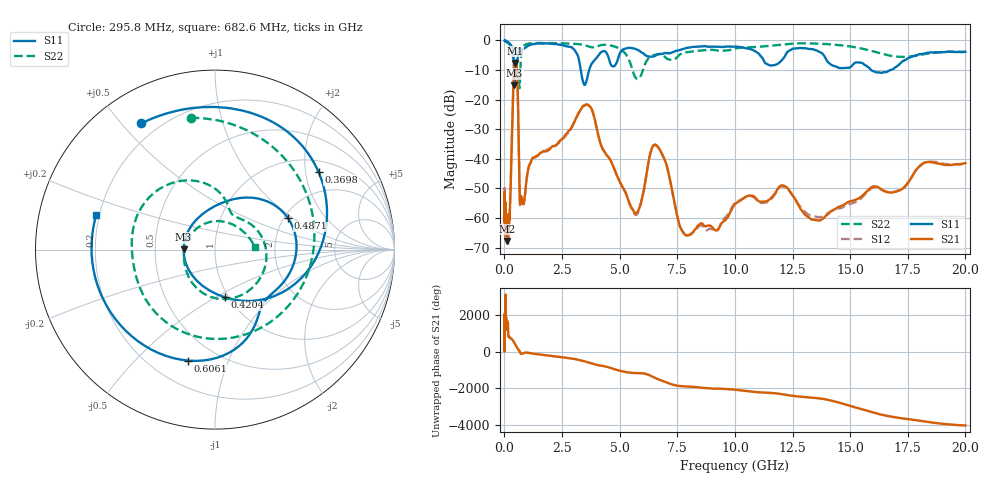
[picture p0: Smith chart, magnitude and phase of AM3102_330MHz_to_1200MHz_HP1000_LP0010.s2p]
! Date/Time: Tue, Sep 11, 2018 5:16 PM
! Network Analyzer: Agilent Technologies E8362B Rev: A.07.50.63
! Sweep from 0.010 to 20.000 GHz, 1601 Points, Sweep Type: LOG
! Power Supply: 4.949 V, 0.001 A
# Hz S DB R 50
!freq MagS11 AngS11 MagS21 AngS21 MagS12 AngS12 MagS22 AngS22
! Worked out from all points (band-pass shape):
!   1601 points, 10 MHz to 20 GHz, reference 50 ohm
!   highest |S21| = -7.59 dB at 455.8 MHz (marker M1); lowest = -67.8 dB at 118.3 MHz (marker M2)
!   |S21| within 3 dB of the highest: 411.3 MHz to 552.9 MHz (141.6 MHz wide, 29.4 % of centre)
!   lowest |S11| = -15.1 dB at 438.8 MHz (marker M3), VSWR 1.42, Z = 35.1 + j0.0801 ohm
!   |S11| at or under -10 dB: 416.7 MHz to 464.2 MHz (47.47 MHz wide, 10.8 % of centre); 3.315 GHz to 3.678 GHz (362.8 MHz wide, 10.4 % of centre); 15.91 GHz to 16.76 GHz (847.6 MHz wide, 5.19 % of centre)
!   |S22| runs from -16.2 to -0.1 dB; largest |S21 - S12| = 0.006
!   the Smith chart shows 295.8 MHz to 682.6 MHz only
!   S11 on the Smith chart (normalised r, x): 295.8 MHz: 0.14, +0.56; 369.8 MHz: 1.31, +2.36; 420.4 MHz: 0.96, -0.55; 487.1 MHz: 2.10, +0.92; 606.1 MHz: 0.35, -0.72; 682.6 MHz: 0.19, +0.14
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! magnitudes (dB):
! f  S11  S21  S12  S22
! 10 MHz  0.0  -61.1  -50.6  -0.1
! 35.55 MHz  0.0  -61.0  -63.9  -0.3
! 118.3 MHz  -0.3  -67.8  -64.3  -0.7
! 126.4 MHz  -0.4  -65.9  -63.6  -0.7
! 211.1 MHz  -1.0  -60.4  -62.5  -1.2
! 295.8 MHz  -1.8  -42.3  -42.3  -2.5
! 369.8 MHz  -2.8  -20.0  -20.0  -5.7
! 420.4 MHz  -11.4  -9.3  -9.4  -6.5
! 438.8 MHz  -15.1  -7.9  -7.9  -6.7
! 447.2 MHz  -14.5  -7.7  -7.7  -6.7
! 455.8 MHz  -12.4  -7.6  -7.7  -6.6
! 487.1 MHz  -7.1  -7.9  -7.9  -6.8
! 606.1 MHz  -3.9  -27.3  -27.4  -10.6
! 682.6 MHz  -3.2  -55.2  -56.0  -13.0
! 1.59 GHz  -1.0  -37.9  -37.9  -0.9
! 3.634 GHz  -11.4  -21.9  -21.7  -2.0
! 5.652 GHz  -2.8  -58.2  -58.7  -12.1
! 6.549 GHz  -5.2  -35.2  -35.4  -4.8
! 7.958 GHz  -2.5  -65.9  -65.8  -3.9
! 12.03 GHz  -6.7  -49.0  -49.4  -1.4
! 13.68 GHz  -3.9  -60.9  -59.7  -1.1
! 20 GHz  -3.9  -41.5  -42.0  -3.8
